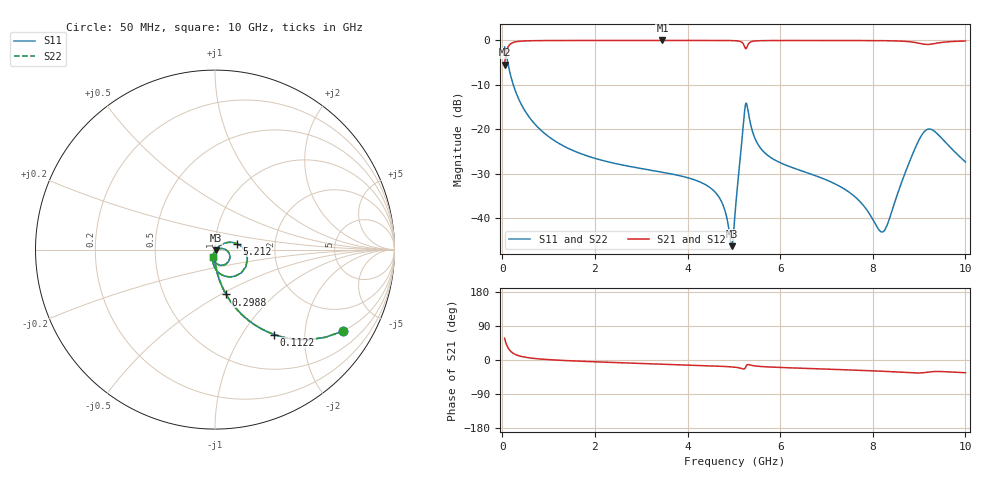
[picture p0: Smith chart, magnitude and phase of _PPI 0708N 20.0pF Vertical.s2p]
! S-Parameter data specifications (vertical orientation):
! Substrate: 40-mil Rogers 3003C, Substrate thickness, H=1.016mm, Dielectric constant, Er=3, Conductor thickness, T_mtl=0.043mm, Loss Tangent, Tand=0.003
! PCB Mounting Pad Footprint: Pad width, PadW=2.54mm , Pad length, PadL=0.51mm , Pad gap, PadG (edge-to-edge)=0.71mm , Reference planes=1.73mm apart
! Created Tue Jan 16 08:52:29 2018
# GHz S MA R 50
! 2 Port Network Data from SP1.SP block
! freq  magS11  angS11  magS21  angS21  magS12  angS12  magS22  angS22
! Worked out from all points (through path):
!   801 points, 50 MHz to 10 GHz, reference 50 ohm
!   highest |S21| = -0.01 dB at 3.458 GHz (marker M1); lowest = -5.5 dB at 50 MHz (marker M2)
!   group delay of S21, straight-line fit = 12.3 ps
!   lowest |S11| = -46.2 dB at 4.95 GHz (marker M3), VSWR 1.01, Z = 50.4 - j0.299 ohm
!   |S11| at or under -10 dB: 238.2 MHz to end of sweep
!   |S22| runs from -46.2 to -1.5 dB; largest |S21 - S12| = 0
!   S11 on the Smith chart (normalised r, x): 50 MHz: 0.99, -3.15; 112.2 MHz: 0.99, -1.40; 298.8 MHz: 0.99, -0.53; 5.212 GHz: 1.27, +0.09; 10 GHz: 0.98, -0.08
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0.05  0.8455 -32.5  0.5339 57.5  0.5339 57.5  0.8455 -32.5
0.1121875  0.5767 -55.2  0.8167 34.8  0.8167 34.8  0.5767 -55.2
0.29875  0.2572 -76.2  0.9661 13.8  0.9661 13.8  0.2572 -76.2
0.821125  0.09935 -87.2  0.9947 2.6  0.9947 2.6  0.09935 -87.2
1.716625  0.05288 -92.9  0.9981 -3.4  0.9981 -3.4  0.05288 -92.9
3.370812  0.03364 -99.5  0.9986 -10.6  0.9986 -10.6  0.03364 -99.5
3.457875  0.03302 -99.8  0.9986 -11.0  0.9986 -11.0  0.03302 -99.8
4.564813  0.02049 -101.9  0.9982 -15.8  0.9982 -15.8  0.02049 -101.9
4.77625  0.01371 -97.5  0.9975 -16.9  0.9975 -16.9  0.01371 -97.5
4.950375  0.004876 -37.5  0.9952 -18.2  0.9952 -18.2  0.004876 -37.5
5.025  0.01121 28.7  0.9922 -19.1  0.9922 -19.1  0.01121 28.7
5.211563  0.1249 15.7  0.9003 -23.8  0.9003 -23.8  0.1249 15.7
5.286187  0.1854 -53.3  0.8519 -12.6  0.8519 -12.6  0.1854 -53.3
5.447875  0.08112 -96.7  0.9842 -15.5  0.9842 -15.5  0.08112 -96.7
5.646875  0.05586 -103.5  0.9942 -17.6  0.9942 -17.6  0.05586 -103.5
6.691625  0.03114 -109.7  0.9976 -22.8  0.9976 -22.8  0.03114 -109.7
7.587125  0.018 -107.7  0.9967 -26.6  0.9967 -26.6  0.018 -107.7
8.171688  0.007107 -57.9  0.9934 -29.5  0.9934 -29.5  0.007107 -57.9
8.345812  0.009458 -11.0  0.9907 -30.5  0.9907 -30.5  0.009458 -11.0
8.830875  0.04849 5.2  0.9614 -33.7  0.9614 -33.7  0.04849 5.2
9.141813  0.09744 -34.4  0.9022 -32.8  0.9022 -32.8  0.09744 -34.4
10  0.04311 -103.3  0.9838 -33.5  0.9838 -33.5  0.04311 -103.3
